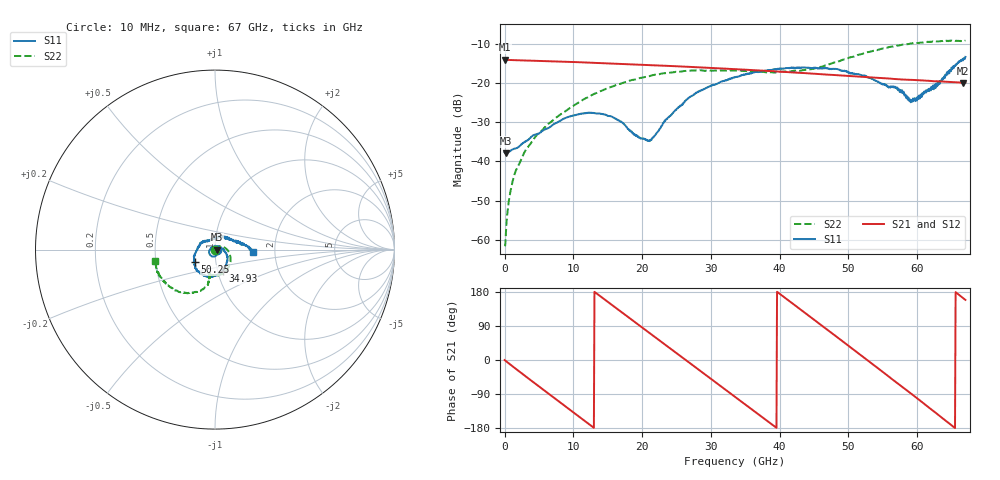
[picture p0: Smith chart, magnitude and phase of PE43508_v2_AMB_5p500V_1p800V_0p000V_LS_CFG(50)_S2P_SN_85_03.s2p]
!Keysight Technologies,N5227A,US51270237,A.10.43.00
!Date: Wednesday, August 22, 2018 17:11:48
!Correction: S11(Full 2 Port(1,3))
!S31(Full 2 Port(1,3))
!S13(Full 2 Port(1,3))
!S33(Full 2 Port(1,3))
!S2P File: Measurements: S11, S31, S13, S33:
# Hz S  dB  R 50
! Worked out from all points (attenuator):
!   801 points, 10 MHz to 67 GHz, reference 50 ohm
!   highest |S21| = -14.13 dB at 10 MHz (marker M1); lowest = -20.0 dB at 66.67 GHz (marker M2)
!   lowest |S11| = -37.9 dB at 261.2 MHz (marker M3), VSWR 1.03, Z = 51.3 - j0.05 ohm
!   |S11| at or under -10 dB: start of sweep to end of sweep
!   |S22| runs from -61.6 to -9.2 dB; largest |S21 - S12| = 0.001
!   S11 on the Smith chart (normalised r, x): 10 MHz: 1.03, -0.00; 34.93 GHz: 1.06, -0.26; 50.25 GHz: 0.79, -0.11; 67 GHz: 1.54, -0.04
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1e7  -37.71 -2.2  -14.13 -0.2  -14.13 -0.2  -61.57 -16.9
2.612125e8  -37.94 -2.2  -14.15 -3.8  -14.16 -3.9  -56.37 58.2
6.799e8  -37.48 -6.4  -14.18 -9.8  -14.18 -9.8  -49.43 64.4
1.182325e9  -36.91 -10.8  -14.21 -16.9  -14.21 -16.9  -45.00 62.9
3.02455e9  -35.00 -27.7  -14.31 -42.6  -14.31 -42.6  -37.28 56.3
6.206575e9  -31.65 -57.5  -14.48 -86.4  -14.48 -86.3  -30.69 40.3
1.123082e10  -27.81 -106.1  -14.78 -155.1  -14.78 -155.0  -24.52 6.8
1.566891e10  -28.66 -153.8  -15.08 144.5  -15.07 144.6  -20.96 -20.9
2.07769e10  -34.52 96.6  -15.45 75.3  -15.44 75.3  -18.39 -49.4
2.236791e10  -32.25 42.7  -15.57 53.7  -15.57 53.7  -17.84 -57.7
2.6806e10  -23.81 -18.3  -15.92 -6.4  -15.92 -6.3  -16.93 -77.4
3.040671e10  -20.56 -44.1  -16.24 -55.1  -16.24 -55.1  -16.90 -90.1
3.3505e10  -18.57 -63.9  -16.52 -97.1  -16.52 -97.1  -16.87 -98.1
3.492854e10  -17.92 -70.2  -16.64 -116.4  -16.65 -116.3  -17.01 -100.3
3.970158e10  -16.40 -95.9  -17.12 178.8  -17.11 178.8  -17.22 -104.5
4.472582e10  -16.22 -120.6  -17.63 110.1  -17.62 110.1  -16.49 -101.2
5.02525e10  -17.65 -147.8  -18.27 34.0  -18.27 34.0  -13.52 -103.3
5.586291e10  -21.20 164.7  -18.88 -43.8  -18.88 -44.2  -10.91 -121.5
5.96311e10  -23.90 99.7  -19.29 -96.1  -19.30 -96.3  -9.94 -135.8
6.29806e10  -19.79 40.5  -19.59 -143.5  -19.61 -143.9  -9.46 -151.0
6.666505e10  -14.28 0.3  -20.00 163.4  -20.07 163.5  -9.33 -166.9
6.7e10  -13.40 -3.0  -19.99 158.6  -20.06 158.6  -9.32 -169.1
